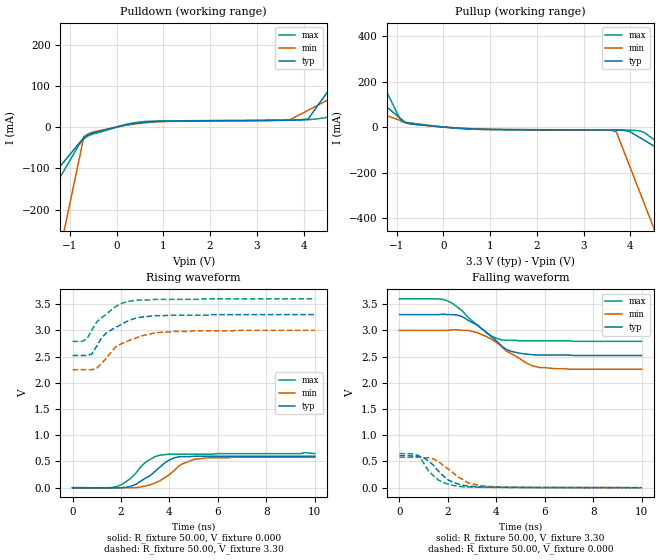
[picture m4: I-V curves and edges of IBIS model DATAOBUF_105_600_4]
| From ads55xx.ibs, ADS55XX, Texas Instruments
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|   Model DATAOBUF_105_600_4
[Model]   DATAOBUF_105_600_4
Model_type   Output
Polarity   Non-Inverting
Vmeas =   1.65V
C_comp   3.00pF   3.00pF   3.00pF
[Temperature Range]   50.00   0.10k   -20.00
[Voltage Range]   3.30V   3.00V   3.60V
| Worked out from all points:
|   slope of the pulldown table from 0 to 0.495 V, typ, clamps not added: 47.8 ohm
|   slope of the pullup table from 0 to 0.495 V, typ, clamps not added: 68.8 ohm
|   rising waveform, R_fixture 50.00, V_fixture 0.000: 20-80 % time 1.03ns typ, 1.05ns min, 876ps max; typ from 0 V to 0.6 V
|   rising waveform, R_fixture 50.00, V_fixture 3.30: 20-80 % time 1.17ns typ, 1.34ns min, 1.01ns max; typ from 2.52 V to 3.3 V
|   falling waveform, R_fixture 50.00, V_fixture 3.30: 20-80 % time 1.27ns typ, 1.43ns min, 1.19ns max; typ from 3.3 V to 2.52 V
|   falling waveform, R_fixture 50.00, V_fixture 0.000: 20-80 % time 880ps typ, 1.04ns min, 748ps max; typ from 0.61 V to 0.001 V
[Pulldown]
| voltage   I(typ)   I(min)   I(max)
-3.3V     -382.8mA   -1.431A    -527.6mA
-2.3V     -245.4mA   -890mA     -333.6mA
-1.9V     -190.4mA   -673.5mA   -255.9mA
-1.5V     -135.5mA   -457mA     -178.3mA
-1V       -66.78mA   -186.3mA   -81.22mA
-700mV    -25.56mA   -23.91mA   -29.24mA
100mV     2.76mA     2.27mA     3.54mA
800mV     13.38mA    12.02mA    14.42mA
3.7V      16.83mA    17.11mA    16.77mA
4.1V      19.69mA    40.83mA    17.84mA
5.5V      241.9mA    123.9mA    40.47mA
6.6V      416.4mA    189.1mA    59.28mA
[Pullup]
| voltage   I(typ)   I(min)   I(max)
-3.3V     446.8mA    201.9mA    1.026A
-3.1V     412.5mA    187.3mA    942.4mA
-1.9V     206.4mA    100.1mA    441.3mA
-900mV    34.75mA    27.39mA    23.66mA
-800mV    17.58mA    20.12mA    20.49mA
500mV     -6.91mA    -6.19mA    -8.28mA
3.6V      -12.54mA   -14.73mA   -13.33mA
3.7V      -12.67mA   -21.32mA   -13.38mA
4V        -21.28mA   -179.5mA   -13.77mA
4.2V      -45.92mA   -285mA     -16.89mA
4.5V      -82.88mA   -443.2mA   -54.27mA
6.6V      -341.6mA   -1.55A     -373.6mA
[Ramp]
| variable   typ   min   max
dV/dt_r   0.36/0.97n   0.35/1.11n   0.39/0.88n
dV/dt_f   0.47/1.29n   0.45/1.43n   0.48/1.17n
R_load = 50.00
[Rising Waveform]
R_fixture = 50.00
V_fixture = 0.000
V_fixture_min = 0.000
V_fixture_max = 0.000
| time   V(typ)   V(min)   V(max)
0s        14.64nV    17.98nV    29.89nV
1.8ns     -2.61mV    -1.48mV    19.01mV
2.2ns     7.77mV     -2.48mV    110mV
2.6ns     60.58mV    120uV      270mV
3ns       180mV      33.15mV    480mV
3.6ns     390mV      130mV      620mV
4.2ns     570mV      330mV      640mV
4.4ns     590mV      420mV      640mV
5ns       600mV      540mV      640mV
10ns      600mV      580mV      650mV
[Rising Waveform]
R_fixture = 50.00
V_fixture = 3.30
V_fixture_min = 3.00
V_fixture_max = 3.60
| time   V(typ)   V(min)   V(max)
0s        2.52V      2.25V      2.79V
600ps     2.52V      2.25V      2.84V
800ps     2.55V      2.25V      3.01V
1ns       2.7V       2.28V      3.16V
1.4ns     2.95V      2.47V      3.31V
1.8ns     3.06V      2.69V      3.46V
2.4ns     3.2V       2.82V      3.56V
3.4ns     3.28V      2.95V      3.59V
4.2ns     3.29V      2.98V      3.59V
10ns      3.3V       3V         3.6V
[Falling Waveform]
R_fixture = 50.00
V_fixture = 3.30
V_fixture_min = 3.00
V_fixture_max = 3.60
| time   V(typ)   V(min)   V(max)
0s        3.3V       3V         3.6V
2ns       3.3V       3V         3.56V
2.6ns     3.26V      3V         3.37V
3.2ns     3.1V       2.96V      3.11V
3.8ns     2.88V      2.83V      2.89V
4.2ns     2.71V      2.7V       2.82V
4.6ns     2.6V       2.56V      2.81V
5.4ns     2.54V      2.34V      2.8V
5.8ns     2.53V      2.29V      2.8V
10ns      2.52V      2.26V      2.79V
[Falling Waveform]
R_fixture = 50.00
V_fixture = 0.000
V_fixture_min = 0.000
V_fixture_max = 0.000
| time   V(typ)   V(min)   V(max)
0s        610mV      580mV      650mV
800ps     600mV      580mV      610mV
1.2ns     510mV      570mV      320mV
1.4ns     430mV      550mV      230mV
1.6ns     320mV      500mV      150mV
2ns       150mV      360mV      69.51mV
2.4ns     74.08mV    210mV      28.73mV
3ns       23.6mV     69.77mV    11.19mV
3.8ns     10.64mV    21.73mV    6.06mV
10ns      1.34mV     1.67mV     1.15mV
